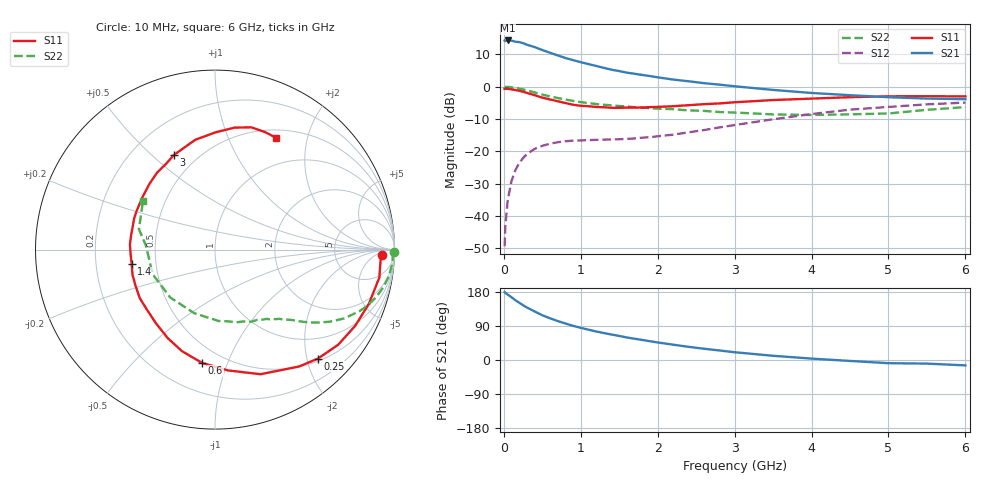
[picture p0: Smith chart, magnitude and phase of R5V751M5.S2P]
! SIEMENS Small Signal Semiconductors
! BFR183
! Si NPN RF Bipolar Junction Transistor in SOT23
! VCE = 0.75 V  IC = 1.5 mA
! Common Emitter S-Parameters:  May  1996
# GHz  S  MA  R  50
!  f  S11  S21  S12  S22
! GHz  MAG  ANG  MAG  ANG  MAG  ANG  MAG  ANG
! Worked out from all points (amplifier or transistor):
!   36 points, 10 MHz to 6 GHz, reference 50 ohm
!   highest |S21| = 14.3 dB at 50 MHz (marker M1)
!   |S21| within 3 dB of that: start of sweep to 504 MHz
!   unconditionally stable (mu >= 1): 1.44 GHz to 3.262 GHz
!   at 250 MHz: K = 0.20, MSG = 17.8 dB, |S12| = -22.1 dB
!   at 1.4 GHz: K = 0.98, MSG = 10.8 dB, |S12| = -16.3 dB
!   at 6 GHz: K = 0.98, MSG = 0.5 dB, |S12| = -4.9 dB
!   S11 on the Smith chart (normalised r, x): 10 MHz: 22, -11; 250 MHz: 0.55, -2.21; 600 MHz: 0.39, -0.82; 1.4 GHz: 0.36, -0.08; 3 GHz: 0.37, +0.59; 6 GHz: 0.60, +1.51
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0.01  0.9291 -2.0  5.193 179.0  0.0034 91.9  0.9954 -0.9
0.02  0.9242 -4.0  5.091 177.0  0.007 88.2  0.9911 -1.7
0.05  0.9289 -9.6  5.202 172.7  0.0174 84.4  0.9914 -4.3
0.1  0.909 -19.4  5.173 165.6  0.0349 78.8  0.9804 -8.6
0.2  0.8672 -37.7  4.908 151.1  0.0658 68.4  0.9361 -16.4
0.25  0.8353 -46.6  4.726 144.5  0.0787 63.4  0.9058 -20.1
0.3  0.8026 -54.2  4.467 138.5  0.0906 59.6  0.877 -22.9
0.4  0.7394 -69.9  4.108 128.1  0.109 52.3  0.8164 -28.0
0.5  0.6769 -83.9  3.697 118.0  0.1216 46.4  0.7558 -32.1
0.6  0.6353 -96.5  3.353 110.1  0.1313 41.8  0.7067 -35.1
0.7  0.5954 -107.9  3.057 102.8  0.1381 38.5  0.6689 -37.4
0.8  0.5592 -118.1  2.783 96.4  0.1432 35.7  0.6336 -39.4
0.9  0.5263 -128.6  2.579 90.2  0.1464 33.8  0.6032 -41.1
1.1  0.4989 -147.2  2.241 80.0  0.1491 32.0  0.5579 -44.4
1.4  0.4714 -170.1  1.835 67.2  0.1524 31.6  0.5153 -48.8
1.7  0.4745 169.4  1.586 56.1  0.1582 34.9  0.4817 -53.3
2.2  0.4983 144.3  1.29 40.4  0.1809 41.1  0.4493 -63.4
3  0.5745 113.6  1.016 20.5  0.255 44.9  0.3983 -87.1
3.5  0.6219 100.1  0.892 11.1  0.3136 41.8  0.3728 -108.0
4.5  0.6882 80.9  0.739 -2.5  0.4419 29.3  0.3736 -158.5
5.5  0.7116 67.1  0.655 -9.5  0.5333 15.0  0.4387 165.0
6  0.7099 61.4  0.642 -14.2  0.5685 6.0  0.4837 146.1
